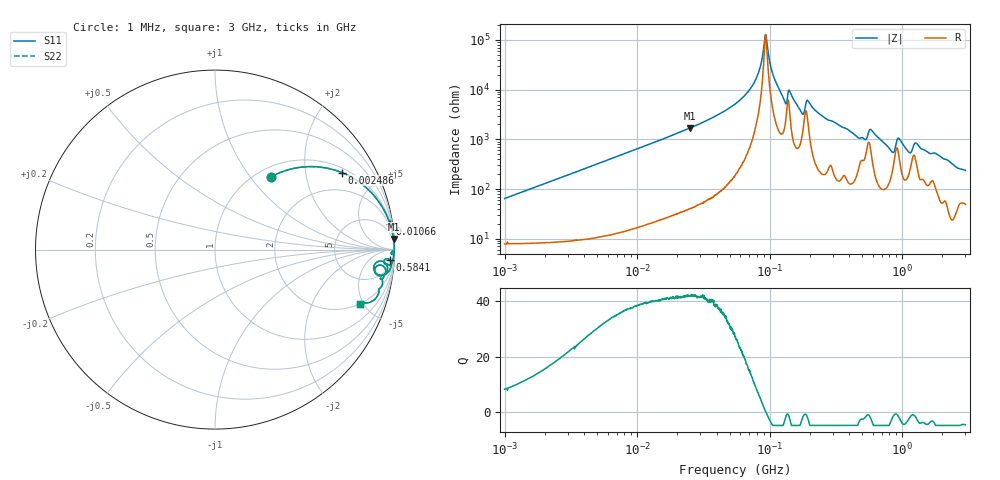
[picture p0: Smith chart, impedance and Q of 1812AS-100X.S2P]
!s-Parameter Generated by FASTRON Sdn. Bhd.
!FASTRON P/N : 1812AS-100X
!Keysight Technologies,E4991B,MY54100416,A.01.15
!Date created: Mon Oct 16 09:32:50 2023
!Version  : Rev00 Mon Oct 16 09:32:50 2023
!Data & Calibration Information:
!Freq	S11	S21	S12	S22
!PortZ  Port1:50+j0  Port2:50+j0
!When reading, reference impedance value at option line is always used.
! Remarks : This data is being provided solely for informational purposes.
# Hz S dB R 50
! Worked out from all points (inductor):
!   1601 points, 1 MHz to 3 GHz, reference 50 ohm
!   read as one part in series: L = 10.2 uH near 1.041 MHz
!   highest Q = 42.2 at 24.97 MHz (marker M1), where L = 10.7 uH
!   self-resonance near 93.09 MHz
!   S11 on the Smith chart (normalised r, x): 1 MHz: 1.16, +1.28; 2.486 MHz: 1.17, +3.17; 10.66 MHz: 1, +14; 584.1 MHz: 11, -29; 3 GHz: 1.98, -4.66
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1000000  -5.79 52.4  -1.96 -30.6  -1.96 -30.6  -5.79 52.4
2486123  -1.66 31.3  -5.67 -55.6  -5.67 -55.6  -1.66 31.3
3804036  -0.80 22.1  -8.50 -65.7  -8.50 -65.7  -0.80 22.1
1.066409e7  -0.12 8.3  -16.81 -80.2  -16.81 -80.2  -0.12 8.3
1.447069e7  -0.07 6.1  -19.47 -82.5  -19.47 -82.5  -0.07 6.1
2.49671e7  -0.03 3.4  -24.53 -85.2  -24.53 -85.2  -0.03 3.4
5.477226e7  -0.01 1.1  -34.19 -86.8  -34.19 -86.8  -0.01 1.1
7.774719e7  -0.01 0.4  -43.61 -83.5  -43.61 -83.5  -0.01 0.4
9.309362e7  -0.01 0.0  -62.22 -6.3  -62.22 -6.3  -0.01 0.0
1.060286e8  -0.01 -0.3  -46.06 78.7  -46.06 78.7  -0.01 -0.3
1.288778e8  -0.04 -0.9  -35.74 74.1  -35.74 74.1  -0.04 -0.9
1.424433e8  -0.03 -0.6  -39.18 70.9  -39.18 70.9  -0.03 -0.6
1.748812e8  -0.09 -1.6  -30.67 69.7  -30.67 69.7  -0.09 -1.6
1.93289e8  -0.06 -0.9  -35.73 64.6  -35.73 64.6  -0.06 -0.9
2.083556e8  -0.03 -1.2  -33.16 81.5  -33.16 81.5  -0.03 -1.2
4.639993e8  -0.20 -5.0  -20.92 72.9  -20.92 72.9  -0.20 -5.0
5.840965e8  -0.20 -3.4  -24.00 67.2  -24.00 67.2  -0.20 -3.4
7.925923e8  -0.32 -8.1  -16.91 71.2  -16.91 71.2  -0.32 -8.1
9.395906e8  -0.42 -4.6  -20.86 56.6  -20.86 56.6  -0.42 -4.6
1.125055e9  -0.66 -9.0  -15.47 59.8  -15.47 59.8  -0.66 -9.0
1.274982e9  -0.46 -5.9  -18.93 60.2  -18.93 60.2  -0.46 -5.9
3e9  -1.30 -20.7  -8.84 57.4  -8.84 57.4  -1.30 -20.7
